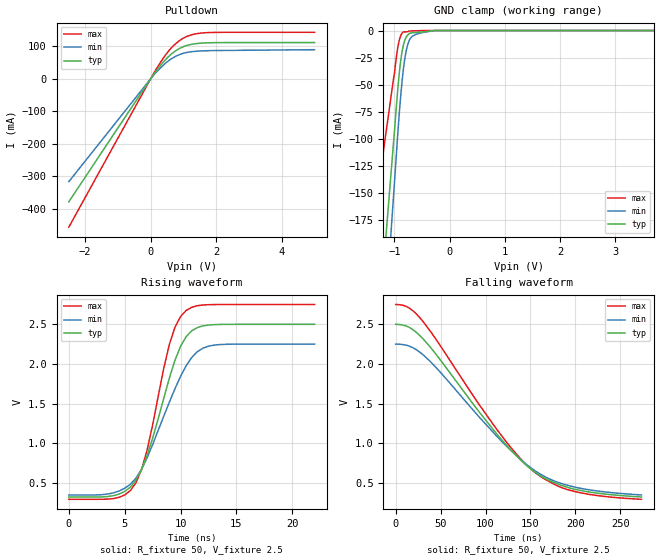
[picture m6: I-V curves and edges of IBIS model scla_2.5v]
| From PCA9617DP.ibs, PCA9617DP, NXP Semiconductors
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[Model]   scla_2.5v
Model_type Open_drain
Vref=2.500E+00
Rref=1.350E+03
Cref=5.000E-11
Vmeas=1.250E+00
C_comp   9.000E-13   8.790E-13   9.210E-13
[Voltage Range]   2.500E+00   2.250E+00   2.750E+00
[POWER Clamp Reference]   2.500E+00   2.250E+00   2.750E+00
[GND Clamp Reference]   0.000E+00   0.000E+00   0.000E+00
[Pullup Reference]   2.500E+00   2.250E+00   2.750E+00
[Pulldown Reference]   0.000E+00   0.000E+00   0.000E+00
[Temperature Range]   25   85   -40
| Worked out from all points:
|   slope of the pulldown table from 0 to 0.375 V, typ, clamps not added: 7.5 ohm
|   GND clamp passes 1 mA (typ) near -0.44 V on its own axis
|   rising waveform, R_fixture 50, V_fixture 2.5: 20-80 % time 2.79ns typ, 3.39ns min, 2.28ns max; typ from 0.321 V to 2.5 V
|   falling waveform, R_fixture 50, V_fixture 2.5: 20-80 % time 93.1ns typ, 94.4ns min, 92.7ns max; typ from 2.5 V to 0.321 V
[GND Clamp]
-2.5V     -1.042A    -1.253A    -587.4mA
-1.02V    -105.8mA   -155.8mA   -45.89mA
-1V       -93.88mA   -141.3mA   -39.77mA
-960mV    -66.98mA   -110.9mA   -22.67mA
-920mV    -43.43mA   -82.02mA   -10.6mA
-880mV    -25.58mA   -56.74mA   -4.036mA
-840mV    -13.98mA   -36.64mA   -1.304mA
-800mV    -7.446mA   -22.27mA   -1.232mA
-760mV    -4.141mA   -13.14mA   -1.161mA
-680mV    -2.023mA   -5.353mA   -333.9uA
-280mV    -71.75uA   -113.6uA   -15.21uA
5V        0A         0A         0A
[Pulldown]
-2.5V     -378.8mA   -316.9mA   -456.9mA
140mV     20.27mA    16.68mA    25.01mA
380mV     50.61mA    41.26mA    62.82mA
540mV     67.68mA    54.85mA    84.43mA
860mV     91.83mA    73.41mA    115.9mA
1.06V     100.9mA    79.82mA    128mA
1.24V     105.7mA    83mA       134.8mA
1.68V     110.2mA    85.97mA    141.5mA
5V        111.2mA    89.22mA    142.7mA
[Rising Waveform]
R_fixture = 50
V_fixture = 2.5
V_fixture_min = 2.25
V_fixture_max = 2.75
0s        321.1mV    346.8mV    291.4mV
4.5ns     357.9mV    396.3mV    316.7mV
6ns       531.3mV    557.6mV    497.7mV
7ns       844.1mV    812.2mV    908.5mV
9ns       1.821V     1.518V     2.246V
9.5ns     2.046V     1.686V     2.462V
10.5ns    2.344V     1.977V     2.674V
11.5ns    2.459V     2.154V     2.734V
13ns      2.496V     2.237V     2.749V
22ns      2.5V       2.25V      2.75V
[Falling Waveform]
R_fixture = 50
V_fixture = 2.5
V_fixture_min = 2.25
V_fixture_max = 2.75
0s        2.5V       2.25V      2.75V
14ns      2.467V     2.229V     2.713V
28.5ns    2.339V     2.134V     2.561V
48ns      2.076V     1.917V     2.258V
112.5ns   1.116V     1.088V     1.174V
135.5ns   826.4mV    830.7mV    847mV
154.5ns   639.2mV    656.2mV    635.2mV
177.5ns   497mV      518.7mV    475.2mV
198ns     422.4mV    449.4mV    393.5mV
273.5ns   321.1mV    346.8mV    291.4mV
[Ramp]
dV/dt_r   1.3073E+00/2.7730E-09   1.1419E+00/3.3730E-09   1.4751E+00/2.2580E-09
dV/dt_f   1.3073E+00/9.3062E-08   1.1419E+00/9.4334E-08   1.4751E+00/9.2669E-08
R_load = 50
